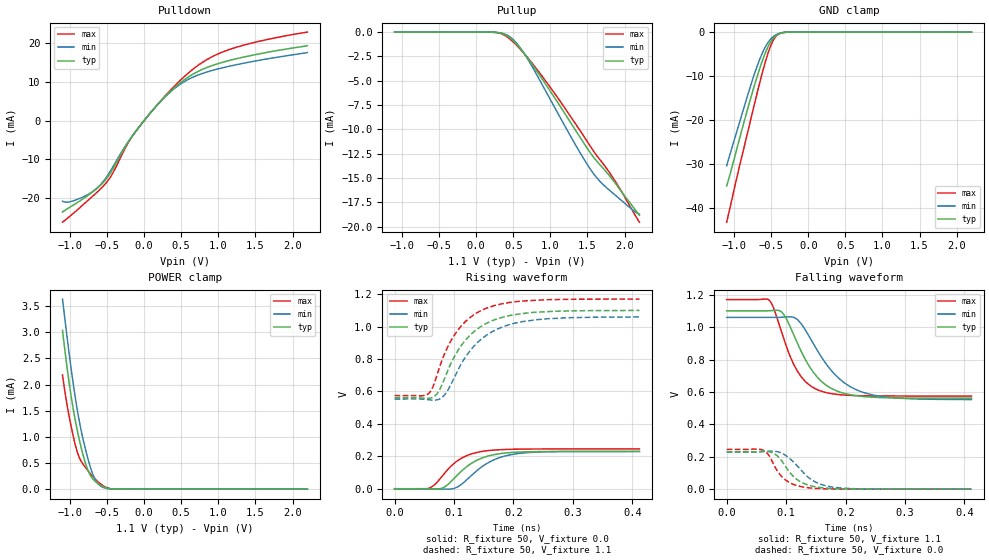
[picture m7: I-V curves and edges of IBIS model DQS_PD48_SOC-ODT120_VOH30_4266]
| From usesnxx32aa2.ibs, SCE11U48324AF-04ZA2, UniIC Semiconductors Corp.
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| DQS_PD48_SOC-ODT120_VOH30_4266
| (48 Ohm Pulldown, 120 Ohm System ODT Setting, VOH=VDDQ/3.0, 3200-4266Mbps)
[Model]   DQS_PD48_SOC-ODT120_VOH30_4266
Model_type   I/O
Vinl = 123.333mV
Vinh = 243.333mV
Vmeas = 183.333mV
Vref = 0.0mV
Cref = 0.0pF
Rref = 120.000Ohm
|   typ   min   max
|C_comp   0.838pF   0.788pF   0.888pF
C_comp_pullup   0.4190pF   0.3940pF   0.4440pF
C_comp_pulldown   0.4190pF   0.3940pF   0.4440pF
| Note: C_comp changes when the ODT circuit is enabled.
[Model Spec]
| Input threshold voltage corners
Vinl   0.1233V   0.1167V   0.1350V
Vinh   0.2433V   0.2367V   0.2550V
| Measurement voltage corners
Vmeas   0.1833V   0.1767V   0.1950V
| Timing spec test load voltage corners
Vref   0.0000V   0.0000V   0.0000V
| Dynamic Overshoot Parameters from LPDDR4 Specification
D_overshoot_ampl_h   0.30   NA   NA
D_overshoot_ampl_l   0.30   NA   NA
D_overshoot_area_h   0.1n   NA   NA
D_overshoot_area_l   0.1n   NA   NA
[Receiver Thresholds]
Vcross_low   = 123.3mV
Vcross_high  = 243.3mV
Vdiff_ac   = 120mV
Vdiff_dc   = 120mV
Tdiffslew_ac = 10.000ns |Not specified, so set to high value
[Voltage Range]   1.1000V   1.0600V   1.1700V
[Pullup Reference]   1.1000V   1.0600V   1.1700V
| Junction Temperature (Ambient temp is 35C typ 95C min -40C max)
[Temperature Range]   50.0   110.0   -40.0
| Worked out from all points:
|   slope of the pulldown table from 0 to 0.165 V, typ, clamps not added: 43.9 ohm
|   slope of the pullup table from 0 to 0.165 V, typ, clamps not added: 38.9 kohm
|   GND clamp passes 1 mA (typ) near -0.45 V on its own axis
|   POWER clamp passes 1 mA (typ) near -0.88 V on its own axis
|   rising waveform, R_fixture 50, V_fixture 0.0: 20-80 % time 48.1ps typ, 52ps min, 43.1ps max; typ from 0 V to 0.23 V
|   falling waveform, R_fixture 50, V_fixture 1.1: 20-80 % time 50.3ps typ, 62.5ps min, 40.2ps max; typ from 1.1 V to 0.561 V
|   rising waveform, R_fixture 50, V_fixture 1.1: 20-80 % time 59ps typ, 63.2ps min, 54.6ps max; typ from 0.561 V to 1.1 V
|   falling waveform, R_fixture 50, V_fixture 0.0: 20-80 % time 33.2ps typ, 40.8ps min, 28.7ps max; typ from 0.231 V to 0 V
[Pulldown]
|   Voltage   I(typ)   I(min)   I(max)
-1.1V     -23.5mA    -20.7mA    -26.1mA
-1.031V   -22.61mA   -20.96mA   -25.04mA
-908.6mV  -21.16mA   -20.31mA   -23.09mA
-628.1mV  -17.3mA    -17.22mA   -18.29mA
-469.7mV  -13.91mA   -13.43mA   -14.95mA
-169.4mV  -4.248mA   -4.232mA   -4.304mA
127.6mV   2.931mA    2.91mA     2.937mA
408.1mV   8.437mA    8.203mA    8.84mA
675.4mV   12.09mA    11.29mA    13.44mA
896.5mV   13.98mA    12.75mA    16.19mA
1.184V    15.6mA     14.1mA     18.46mA
2.2V      19.2mA     17.45mA    22.72mA
[GND Clamp]
|   Voltage   I(typ)   I(min)   I(max)
-1.1V     -34.88mA   -30.34mA   -43.13mA
-948.2mV  -25.55mA   -21.71mA   -31.95mA
-796.4mV  -16.18mA   -13.19mA   -21.29mA
-720.5mV  -11.79mA   -9.217mA   -15.95mA
-661.1mV  -8.597mA   -6.455mA   -11.9mA
-588.5mV  -5.129mA   -3.689mA   -7.329mA
-522.5mV  -2.67mA    -1.907mA   -3.823mA
-466.4mV  -1.296mA   -944.9uA   -1.694mA
-413.6mV  -566.1uA   -418.5uA   -621.9uA
-344.3mV  -143.3uA   -109.5uA   -124.7uA
-242mV    -9.986uA   -9.216uA   -5.624uA
2.2V      0A         0A         0A
[Pullup]
|   Voltage   I(typ)   I(min)   I(max)
-1.1V     2.095uA    3.229uA    944.4nA
229.9mV   -15.06uA   -15.37uA   -15.54uA
345.4mV   -134.6uA   -110.6uA   -185.9uA
441.1mV   -502uA     -412uA     -628.6uA
556.6mV   -1.343mA   -1.244mA   -1.449mA
688.6mV   -2.62mA    -2.707mA   -2.588mA
1.055V    -6.724mA   -7.711mA   -6.28mA
1.362V    -10.36mA   -11.9mA    -9.692mA
1.556V    -12.6mA    -14.28mA   -11.94mA
1.698V    -13.89mA   -15.58mA   -13.41mA
1.867V    -15.45mA   -16.71mA   -15.25mA
2.2V      -18.83mA   -18.71mA   -19.54mA
[POWER Clamp]
|   Voltage   I(typ)   I(min)   I(max)
-1.1V     3.036mA    3.636mA    2.186mA
-1.044V   2.383mA    2.969mA    1.653mA
-977.9mV  1.724mA    2.242mA    1.161mA
-911.9mV  1.201mA    1.611mA    764.9uA
-852.5mV  818.5uA    1.149mA    543.7uA
-779.9mV  448.2uA    701.7uA    396.3uA
-710.6mV  232.2uA    359.3uA    273.1uA
-654.5mV  142.7uA    170.4uA    185.9uA
-598.4mV  83.7uA     71.97uA    113uA
-489.5mV  17.77uA    10.87uA    22.46uA
-374mV    1.382uA    999.2nA    1.121uA
2.2V      0A         0A         0A
[Ramp]
|   typ   min   max
| 20% - 80%
dV/dt_r   138.15m/48.10p   137.75m/52.05p   147.35m/43.12p
dV/dt_f   323.20m/50.32p   304.17m/62.52p   357.16m/40.16p
| 25% - 75%
|dV/dt_r   115.12m/38.35p   114.79m/41.61p   122.79m/34.20p
|dV/dt_f   269.33m/40.10p   253.48m/49.87p   297.63m/32.01p
R_load = 50
[Rising Waveform]
R_fixture = 50
V_fixture = 0.0
|   Time   V(typ)   V(min)   V(max)
0s        187.1uV    147uV      136.9uV
57ps      -121.9uV   387.8uV    2.281mV
68ps      -1.493mV   -461.1uV   27.72mV
79ps      2.613mV    -1.73mV    72.97mV
106ps     85.81mV    11.51mV    173mV
127ps     151.3mV    74.67mV    212.2mV
148ps     190.7mV    138.7mV    230.8mV
178ps     216.9mV    193.7mV    241.1mV
218ps     227.5mV    221.1mV    244.8mV
412ps     230.4mV    229.7mV    245.7mV
[Falling Waveform]
R_fixture   = 50
V_fixture   = 1.1
V_fixture_min = 1.06
V_fixture_max = 1.17
|   Time   V(typ)   V(min)   V(max)
0s        1.1V       1.06V      1.17V
72ps      1.101V     1.06V      1.165V
93ps      1.091V     1.061V     962.1mV
114ps     942.5mV    1.058V     761.6mV
131ps     809.6mV    990.7mV    669.6mV
154ps     685.3mV    846.9mV    611.7mV
188ps     602.2mV    686.6mV    583.8mV
229ps     571.9mV    597.9mV    576.4mV
288ps     562.8mV    561.7mV    574.9mV
412ps     561.3mV    553mV      574.7mV
[Rising Waveform]
R_fixture   = 50
V_fixture   = 1.1
V_fixture_min = 1.06
V_fixture_max = 1.17
|   Time   V(typ)   V(min)   V(max)
0s        561.2mV    552.6mV    574.7mV
56ps      557.6mV    548.9mV    583.5mV
65ps      565.3mV    546.3mV    633mV
79ps      635.6mV    560.9mV    785.3mV
94ps      766.7mV    637.7mV    907.6mV
112ps     882mV      769.7mV    1.004V
154ps     1.019V     945.6mV    1.113V
190ps     1.065V     1.009V     1.147V
234ps     1.088V     1.041V     1.162V
412ps     1.1V       1.06V      1.17V
[Falling Waveform]
R_fixture = 50
V_fixture = 0.0
|   Time   V(typ)   V(min)   V(max)
0s        230.5mV    229.8mV    245.8mV
58ps      233.2mV    230.7mV    244.9mV
68ps      233.2mV    233.5mV    222.7mV
76ps      226.6mV    234.7mV    176.1mV
97ps      151.2mV    213.7mV    62.59mV
113ps     76.18mV    165.6mV    28.51mV
131ps     33.5mV     94.01mV    11.87mV
154ps     11.89mV    36.36mV    3.974mV
189ps     2.676mV    8.363mV    875.2uV
412ps     263.4uV    253.4uV    169.3uV
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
